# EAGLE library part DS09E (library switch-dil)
DIL/CODE SWITCH
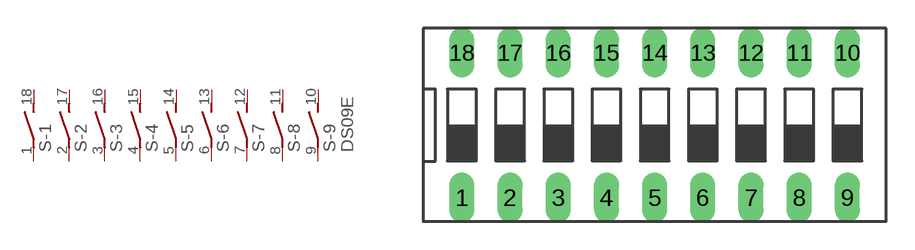
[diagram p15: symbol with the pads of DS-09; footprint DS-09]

Designator prefix S; gates -1=S -2=S -3=S -4=S -5=S -6=S -7=S -8=S -9=S+V

## DS09E (MPN: MCDS09; OC_FARNELL: 1255227; OC_NEWARK: 26M1107)  [DS-09]
1  -1:1  pas
2  -2:1  pas
3  -3:1  pas
4  -4:1  pas
5  -5:1  pas
6  -6:1  pas
7  -7:1  pas
8  -8:1  pas
9  -9:1  pas
10  -9:2  pas
11  -8:2  pas
12  -7:2  pas
13  -6:2  pas
14  -5:2  pas
15  -4:2  pas
16  -3:2  pas
17  -2:2  pas
18  -1:2  pas

## Footprint DS-09 (pad centres in mm)
DIL/CODE SWITCH Mors distributor Buerklin, 17G564
drill 0.813 long: 1 -10.16,-3.81; 2 -7.62,-3.81; 3 -5.08,-3.81; 4 -2.54,-3.81; 5 0,-3.81; 6 2.54,-3.81; 7 5.08,-3.81; 8 7.62,-3.81; 9 10.16,-3.81; 10 10.16,3.81; 11 7.62,3.81; 12 5.08,3.81; 13 2.54,3.81; 14 0,3.81; 15 -2.54,3.81; 16 -5.08,3.81; 17 -7.62,3.81; 18 -10.16,3.81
